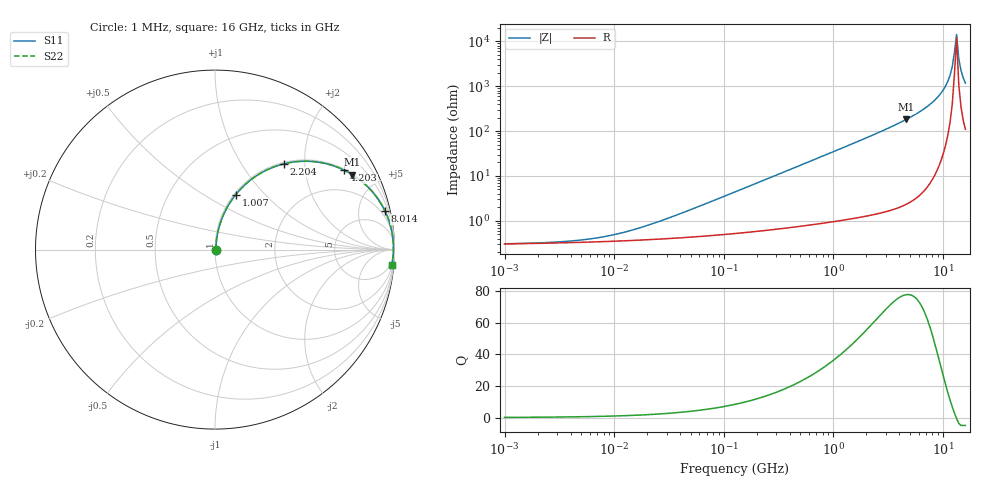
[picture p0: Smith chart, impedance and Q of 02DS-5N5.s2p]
# MHz S MA R 50
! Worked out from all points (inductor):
!   211 points, 1 MHz to 16 GHz, reference 50 ohm
!   read as one part in series: L = 5.5 nH near 36.44 MHz
!   highest Q = 77.8 at 4.609 GHz (marker M1), where L = 6.26 nH
!   self-resonance near 12.71 GHz
!   S11 on the Smith chart (normalised r, x): 1 MHz: 1.01, +0.00; 1.007 GHz: 1.02, +0.70; 2.204 GHz: 1.03, +1.57; 4.203 GHz: 1.04, +3.23; 8.014 GHz: 1.17, +8.77; 16 GHz: 3, -23
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1  0.00307 6.4  0.9969 -0.0  0.9969 -0.0  0.00307 6.4
5.25662  0.003782 28.5  0.9967 -0.1  0.9967 -0.1  0.003782 28.5
11.5091  0.00532 47.9  0.9964 -0.2  0.9964 -0.2  0.00532 47.9
26.3872  0.00989 66.2  0.996 -0.5  0.996 -0.5  0.00989 66.2
132.458  0.04579 80.8  0.9937 -2.6  0.9937 -2.6  0.04579 80.8
318.018  0.1088 80.3  0.9876 -6.2  0.9876 -6.2  0.1088 80.3
664.915  0.2229 75.1  0.9669 -12.9  0.9669 -12.9  0.2229 75.1
1006.8  0.3276 69.3  0.9359 -19.1  0.9359 -19.1  0.3276 69.3
2204.33  0.6118 51.3  0.7806 -37.7  0.7806 -37.7  0.6118 51.3
3187.38  0.7549 40.2  0.6453 -49.0  0.6453 -49.0  0.7549 40.2
4202.92  0.8455 31.5  0.5231 -57.7  0.5231 -57.7  0.8455 31.5
4608.83  0.871 28.7  0.4801 -60.6  0.4801 -60.6  0.871 28.7
6363.96  0.9401 19.1  0.328 -70.0  0.328 -70.0  0.9401 19.1
8013.56  0.971 12.8  0.2213 -76.1  0.2213 -76.1  0.971 12.8
10090.8  0.9885 6.8  0.1178 -81.0  0.1178 -81.0  0.9885 6.8
11587.3  0.9933 3.3  0.05701 -81.6  0.05701 -81.6  0.9933 3.3
12134  0.994 2.1  0.03701 -79.6  0.03701 -79.6  0.994 2.1
12706.4  0.9942 0.9  0.01744 -70.1  0.01744 -70.1  0.9942 0.9
13305.8  0.994 -0.2  0.006995 30.7  0.006995 30.7  0.994 -0.2
13933.5  0.9933 -1.4  0.02452 73.5  0.02452 73.5  0.9933 -1.4
14590.9  0.9922 -2.5  0.04428 78.6  0.04428 78.6  0.9922 -2.5
16000  0.9886 -4.8  0.08434 79.8  0.08434 79.8  0.9886 -4.8
